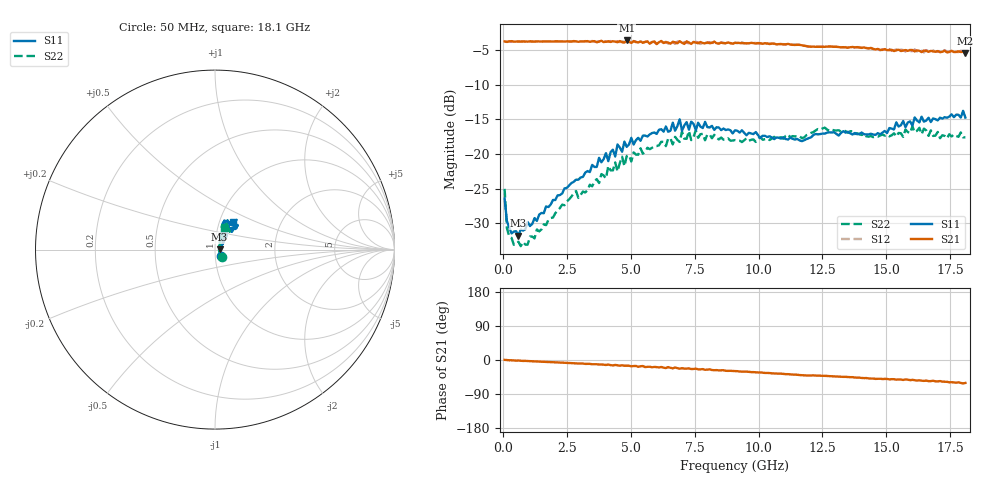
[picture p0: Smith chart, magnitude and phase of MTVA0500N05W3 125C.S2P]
! Network Analyzer HP8720D.06.14 Serial No. US36140669
!  8 Jul 2005  09:23:20
! Frequency  S11  S21  S12  S22
# HZ  S  DB R 50
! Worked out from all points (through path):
!   201 points, 50 MHz to 18.1 GHz, reference 50 ohm
!   highest |S21| = -3.61 dB at 4.833 GHz (marker M1); lowest = -5.4 dB at 18.1 GHz (marker M2)
!   group delay of S21, straight-line fit = 9.43 ps
!   lowest |S11| = -31.8 dB at 591.5 MHz (marker M3), VSWR 1.05, Z = 52.6 + j0.175 ohm
!   |S11| at or under -10 dB: start of sweep to end of sweep
!   |S22| runs from -33.3 to -16.0 dB; largest |S21 - S12| = 0.028
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5e7  -26.41 -48.2  -3.75 0.4  -3.76 0.6  -25.01 -45.6
1.4025e8  -29.67 -29.9  -3.82 -0.2  -3.81 -0.3  -30.68 -32.9
4.11e8  -31.18 -7.0  -3.79 -1.2  -3.77 -1.3  -33.08 -6.4
5.915e8  -31.75 3.7  -3.74 -1.4  -3.79 -1.5  -32.63 5.9
9.525e8  -29.78 16.2  -3.78 -2.8  -3.73 -2.9  -33.05 19.0
3.1185e9  -23.29 46.9  -3.75 -9.2  -3.78 -9.6  -25.39 60.0
4.021e9  -19.86 53.7  -3.78 -13.1  -3.78 -12.2  -23.51 62.3
4.11125e9  -21.02 54.0  -3.73 -12.1  -3.81 -13.2  -21.71 62.9
4.47225e9  -18.61 51.9  -3.87 -14.1  -3.71 -13.6  -22.49 68.9
4.83325e9  -18.96 62.2  -3.61 -15.2  -3.80 -15.7  -20.28 59.9
6.09675e9  -16.48 61.3  -3.86 -19.7  -3.77 -19.5  -18.73 64.4
6.7285e9  -16.62 68.6  -3.88 -19.7  -4.10 -20.5  -17.51 61.2
6.909e9  -14.98 66.9  -3.72 -23.0  -3.81 -21.5  -18.24 61.2
6.99925e9  -16.64 66.7  -3.95 -21.5  -4.09 -23.2  -16.76 62.7
7.36025e9  -15.32 63.2  -4.11 -23.9  -3.85 -23.1  -17.98 66.7
7.54075e9  -16.54 65.6  -3.91 -22.7  -3.80 -25.1  -16.55 65.7
7.90175e9  -15.35 69.5  -4.03 -25.9  -3.92 -24.6  -18.00 61.7
9.075e9  -16.57 71.7  -3.96 -29.3  -3.93 -29.3  -17.98 57.5
1.21435e10  -17.24 63.3  -4.50 -40.6  -4.46 -40.8  -16.83 65.0
1.512175e10  -16.24 49.0  -5.00 -51.2  -4.86 -50.6  -17.43 70.6
1.602425e10  -15.89 47.9  -4.99 -52.4  -5.14 -54.4  -15.99 65.6
1.81e10  -14.73 57.0  -5.39 -60.6  -5.54 -61.6  -17.57 68.4
